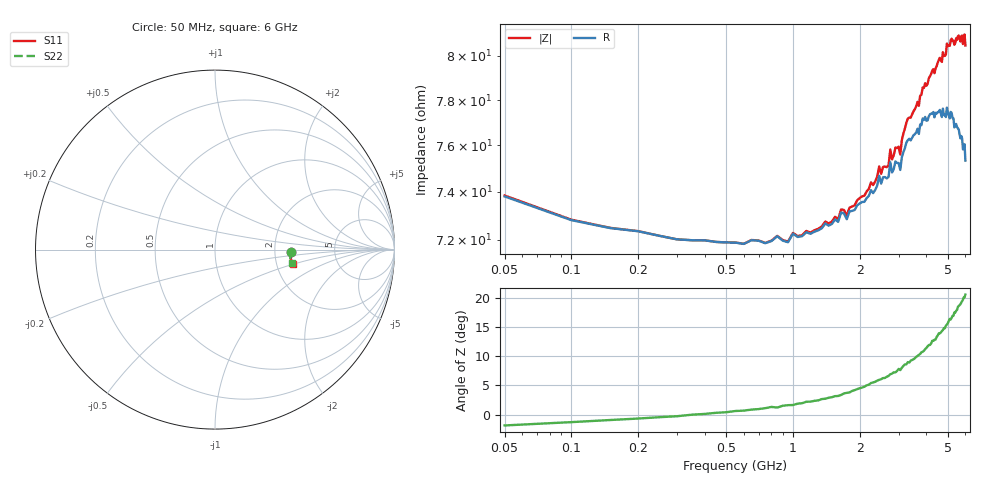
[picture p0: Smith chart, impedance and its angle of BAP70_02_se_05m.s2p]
!	Created	by	janssen	on	Thu	Dec	12	13:21:17	MET	2002
#	HZ	S	MA	R	50
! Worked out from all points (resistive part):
!   120 points, 50 MHz to 6 GHz, reference 50 ohm
!   read as one part in series: R = 73.8 ohm at 50 MHz
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5e7  0.4258 -1.5  0.5756 0.6  0.5751 0.6  0.4246 -1.5
1e8  0.4215 -1.4  0.579 0.2  0.5785 0.2  0.4224 -1.4
2.5e8  0.4197 -1.7  0.5811 -0.6  0.5814 -0.6  0.4197 -1.8
1.05e9  0.4221 -4.9  0.5822 -3.9  0.5824 -3.8  0.4212 -5.1
2.05e9  0.4293 -8.5  0.5773 -7.8  0.579 -7.7  0.4286 -8.8
2.45e9  0.4334 -9.7  0.5727 -9.3  0.5762 -9.2  0.432 -9.6
2.65e9  0.4339 -10.0  0.5739 -9.9  0.5759 -9.9  0.4336 -10.1
2.75e9  0.4365 -9.9  0.5707 -10.3  0.5747 -10.3  0.4342 -10.3
3e9  0.4369 -10.5  0.5708 -11.2  0.5745 -11.2  0.4348 -10.6
3.05e9  0.4382 -11.0  0.5728 -11.3  0.5748 -11.2  0.4343 -11.0
3.1e9  0.4385 -10.8  0.5706 -11.5  0.5719 -11.6  0.4361 -10.8
3.3e9  0.4403 -10.9  0.5672 -12.4  0.5715 -12.2  0.4388 -10.9
3.55e9  0.4419 -11.5  0.5662 -13.1  0.5699 -13.1  0.4398 -11.1
4.05e9  0.4448 -11.4  0.5638 -14.7  0.5669 -14.6  0.4426 -11.2
4.4e9  0.4461 -11.7  0.5614 -15.6  0.566 -15.7  0.4422 -11.1
4.55e9  0.4458 -11.5  0.5602 -16.3  0.5671 -16.6  0.4423 -10.8
4.6e9  0.4465 -11.6  0.5602 -16.4  0.5652 -16.4  0.4431 -11.0
4.9e9  0.4455 -11.7  0.5602 -17.4  0.565 -17.5  0.442 -10.9
5.05e9  0.4467 -11.2  0.5594 -17.9  0.5654 -18.1  0.4421 -10.7
5.6e9  0.4469 -11.0  0.5598 -19.7  0.5641 -19.8  0.4406 -10.2
5.85e9  0.444 -10.7  0.563 -20.2  0.5671 -20.9  0.4411 -9.8
6e9  0.4448 -10.7  0.5636 -20.9  0.5668 -21.3  0.4376 -9.7
